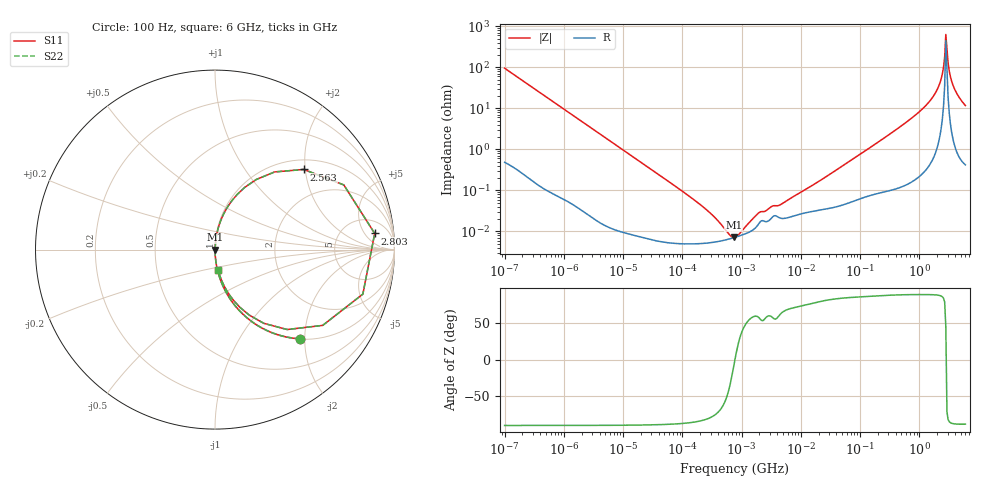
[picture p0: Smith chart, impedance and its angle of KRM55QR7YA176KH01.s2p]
!Murata Part Number: KRM55QR7YA176KH01
!These Parameters are Measured in Series Mode Connection
!Data Generated on Jan 08, 2026
!  o--ll--o
!Port1  Port2
!  o------o
!Operation Temp=25[degC], DC Bias Voltage=0[V]
!Freq. Start=100[Hz] Stop=6[GHz] 401[Steps]
# Hz S RI R 50
!Freq.(Hz) S11(Real) S11(Imag) S21(Real) S21(Imag) S12(Real) S12(Imag) S22(Real) S22(Imag)
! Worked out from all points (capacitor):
!   401 points, 100 Hz to 6 GHz, reference 50 ohm
!   read as one part in series: C = 16.7 uF near 109 Hz
!   lowest |Z| = 7.13 mohm at 740.7 kHz (marker M1)
!   series resonance near 772.7 kHz, so ESL is about 2.5 nH
!   S11 on the Smith chart (normalised r, x): 100 Hz: 1.01, -1.90; 2.563 GHz: 1.22, +1.96; 2.803 GHz: 10, +9; 6 GHz: 1.01, -0.23
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100  0.4747 -0.4968  0.5253 0.4968  0.5253 0.4968  0.4747 -0.4968
320  0.0828 -0.273  0.9172 0.273  0.9172 0.273  0.0828 -0.273
2008  0.00261 -0.0477  0.9974 0.0477  0.9974 0.0477  0.00261 -0.0477
40335  6.31e-05 -0.0024  0.9999 0.0024  0.9999 0.0024  6.31e-05 -0.0024
231233  5.14e-05 -0.000379  0.9999 0.000379  0.9999 0.000379  5.14e-05 -0.000379
541393  6.24e-05 -8.73e-05  0.9999 8.73e-05  0.9999 8.73e-05  6.24e-05 -8.73e-05
740679  7.06e-05 -1e-05  0.9999 1e-05  0.9999 1e-05  7.06e-05 -1e-05
774597  7.2e-05 6e-07  0.9999 -6e-07  0.9999 -6e-07  7.2e-05 6e-07
1013323  8.17e-05 6.33e-05  0.9999 -6.33e-05  0.9999 -6.33e-05  8.17e-05 6.33e-05
1983483  0.000159 0.000242  0.9998 -0.000242  0.9998 -0.000242  0.000159 0.000242
1.555665e7  0.000308 0.00128  0.9997 -0.00128  0.9997 -0.00128  0.000308 0.00128
3.124326e8  0.00152 0.0231  0.9985 -0.0231  0.9985 -0.0231  0.00152 0.0231
1.000774e9  0.00887 0.0815  0.9911 -0.0815  0.9911 -0.0815  0.00887 0.0815
1.791126e9  0.0494 0.201  0.9506 -0.201  0.9506 -0.201  0.0494 0.201
2.240541e9  0.165 0.3461  0.835 -0.3461  0.835 -0.3461  0.165 0.3461
2.450438e9  0.3326 0.4328  0.6674 -0.4328  0.6674 -0.4328  0.3326 0.4328
2.562649e9  0.4948 0.4464  0.5052 -0.4464  0.5052 -0.4464  0.4948 0.4464
2.802721e9  0.8898 0.0898  0.1102 -0.0898  0.1102 -0.0898  0.8898 0.0898
3.065283e9  0.6001 -0.4223  0.3999 0.4223  0.3999 0.4223  0.6001 -0.4223
3.352442e9  0.2719 -0.4107  0.7281 0.4107  0.7281 0.4107  0.2719 -0.4107
4.009986e9  0.0811 -0.2533  0.9189 0.2533  0.9189 0.2533  0.0811 -0.2533
6e9  0.0174 -0.114  0.9826 0.114  0.9826 0.114  0.0174 -0.114
